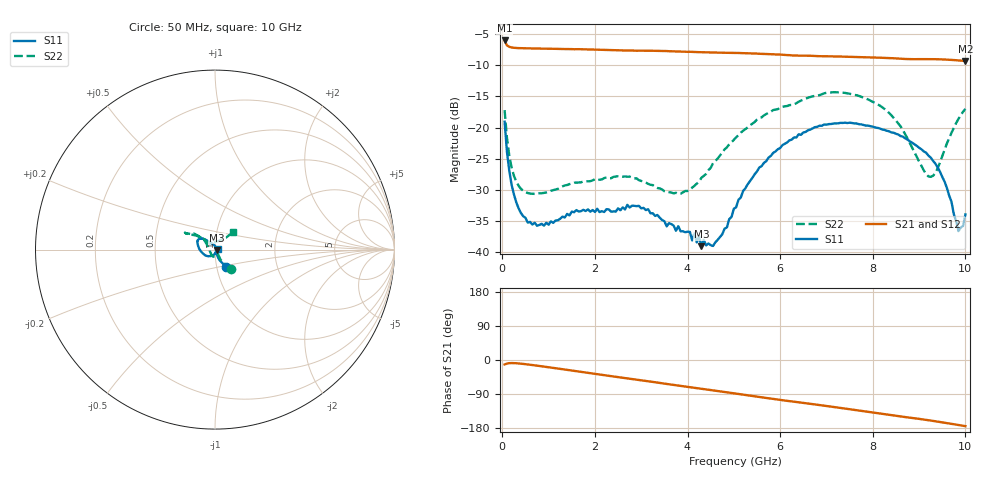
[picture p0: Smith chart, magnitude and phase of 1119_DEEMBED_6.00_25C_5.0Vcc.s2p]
!Hittite Microwave Corp.
!Digital Attenuator/PhaseShifter Rev 1.4.0
!Filename: C:\DATA\DATA\1119_DEEMBED_6.00_25C_5.0Vcc.s2p
!VNA ID: Agilent Technologies,N5224A,MY51441122,A.10.45.03
!Device type:
!2 Port Calibration.
!Temp(C): 25
!Lot Number:
!Serial Number:
!Operator:
!Misc:
!Attenuator:  6.000
# GHZ S DB R 50.0
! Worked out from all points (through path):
!   200 points, 50 MHz to 10 GHz, reference 50 ohm
!   highest |S21| = -6.00 dB at 50 MHz (marker M1); lowest = -9.3 dB at 10 GHz (marker M2)
!   group delay of S21, straight-line fit = 47.2 ps
!   lowest |S11| = -39.1 dB at 4.3 GHz (marker M3), VSWR 1.02, Z = 51.1 - j0.136 ohm
!   |S11| at or under -10 dB: start of sweep to end of sweep
!   |S22| runs from -30.7 to -14.3 dB; largest |S21 - S12| = 0.0014
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0.05  -19.05 -57.6  -6.00 -11.8  -6.00 -11.8  -17.19 -49.9
0.1  -23.88 -66.8  -6.79 -9.5  -6.78 -9.5  -21.60 -59.4
0.2  -29.17 -68.9  -7.12 -8.1  -7.12 -8.1  -26.39 -60.4
0.35  -32.94 -64.7  -7.23 -9.0  -7.23 -9.1  -29.32 -56.0
0.55  -35.27 -63.7  -7.27 -11.7  -7.27 -11.8  -30.52 -54.8
1  -35.61 -73.4  -7.33 -19.1  -7.33 -19.1  -30.30 -62.5
1.75  -33.22 -86.9  -7.42 -32.1  -7.42 -32.1  -28.65 -78.8
2.95  -32.58 -76.0  -7.64 -52.6  -7.65 -52.6  -28.45 -117.1
3.4  -34.49 -67.2  -7.68 -60.4  -7.69 -60.5  -29.77 -134.4
3.85  -36.66 -41.6  -7.78 -68.4  -7.79 -68.4  -30.64 -160.3
4.25  -37.46 -10.2  -7.88 -75.2  -7.90 -75.3  -28.70 168.0
4.3  -39.06 -6.9  -7.89 -76.0  -7.91 -76.1  -28.07 163.7
4.55  -39.03 31.7  -7.93 -80.2  -7.95 -80.3  -25.73 150.5
5.05  -32.80 97.0  -8.01 -88.7  -8.03 -88.8  -21.57 138.6
5.75  -24.82 128.2  -8.20 -101.0  -8.21 -101.1  -17.61 141.7
6.7  -20.13 141.1  -8.48 -116.5  -8.49 -116.5  -14.98 149.2
7.65  -19.34 156.2  -8.66 -132.4  -8.68 -132.4  -14.80 150.9
8.35  -20.59 170.7  -8.83 -144.6  -8.84 -144.6  -17.63 143.2
9.25  -24.81 -141.9  -9.00 -159.8  -9.03 -159.8  -27.92 105.1
9.55  -28.67 -114.7  -9.06 -165.6  -9.08 -165.6  -23.55 55.9
9.85  -36.64 -46.5  -9.20 -171.6  -9.22 -171.6  -18.61 45.1
10  -33.95 14.4  -9.30 -174.6  -9.31 -174.6  -17.00 44.0
